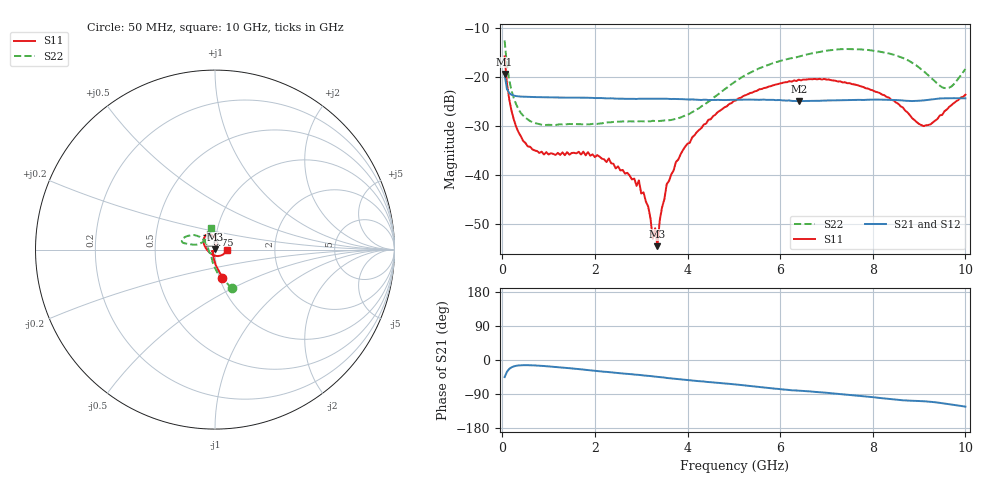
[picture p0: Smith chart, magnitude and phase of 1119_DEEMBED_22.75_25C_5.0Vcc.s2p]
!Hittite Microwave Corp.
!Digital Attenuator/PhaseShifter Rev 1.4.0
!Filename: C:\DATA\DATA\1119_DEEMBED_22.75_25C_5.0Vcc.s2p
!VNA ID: Agilent Technologies,N5224A,MY51441122,A.10.45.03
!Device type:
!2 Port Calibration.
!Temp(C): 25
!Lot Number:
!Serial Number:
!Operator:
!Misc:
!Attenuator:  22.750
# GHZ S DB R 50.0
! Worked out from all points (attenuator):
!   200 points, 50 MHz to 10 GHz, reference 50 ohm
!   highest |S21| = -19.44 dB at 50 MHz (marker M1); lowest = -25.0 dB at 6.4 GHz (marker M2)
!   lowest |S11| = -54.5 dB at 3.35 GHz (marker M3), VSWR 1.00, Z = 49.9 + j0.176 ohm
!   |S11| at or under -10 dB: start of sweep to end of sweep
!   |S22| runs from -29.8 to -12.6 dB; largest |S21 - S12| = 0.00016
!   S11 on the Smith chart (normalised r, x): 50 MHz: 1.03, -0.33; 6.75 GHz: 0.90, +0.15; 10 GHz: 1.14, -0.01
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0.05  -15.83 -75.3  -19.44 -45.1  -19.45 -45.1  -12.60 -66.6
0.1  -21.34 -87.5  -22.49 -31.2  -22.48 -31.2  -17.56 -83.5
0.2  -26.97 -99.7  -23.67 -19.3  -23.68 -19.2  -22.84 -100.2
0.45  -33.09 -117.7  -24.06 -13.7  -24.06 -13.7  -27.92 -120.8
0.9  -35.84 -137.5  -24.17 -15.9  -24.17 -15.9  -29.82 -135.1
1.75  -35.25 -145.1  -24.27 -25.3  -24.27 -25.3  -29.67 -139.8
2.95  -41.13 -130.7  -24.48 -39.3  -24.49 -39.4  -29.08 -158.8
3.15  -46.46 -133.5  -24.49 -41.7  -24.49 -41.8  -29.08 -164.8
3.25  -53.04 -163.3  -24.46 -43.2  -24.47 -43.2  -28.97 -167.5
3.3  -50.88 163.5  -24.48 -43.9  -24.49 -43.9  -29.03 -169.2
3.35  -54.53 109.9  -24.49 -44.5  -24.50 -44.5  -29.07 -170.8
3.4  -49.27 126.3  -24.48 -45.0  -24.49 -45.1  -29.01 -172.2
3.55  -41.89 90.1  -24.48 -47.4  -24.48 -47.4  -28.91 -177.6
3.9  -34.94 77.1  -24.57 -51.8  -24.58 -51.8  -28.11 168.1
5.05  -24.82 87.1  -24.70 -64.6  -24.71 -64.7  -20.85 139.4
6.4  -20.59 111.5  -24.96 -80.8  -24.97 -80.9  -15.90 150.6
6.7  -20.50 117.8  -24.88 -83.6  -24.90 -83.5  -15.20 154.5
6.75  -20.44 118.2  -24.89 -84.1  -24.90 -84.1  -15.12 155.1
8.35  -24.26 160.3  -24.71 -102.7  -24.71 -102.7  -15.25 168.2
9.1  -30.06 -125.9  -24.82 -108.9  -24.83 -108.9  -18.88 166.2
9.6  -26.67 -44.9  -24.38 -115.9  -24.39 -115.8  -22.32 133.3
10  -23.66 -2.1  -24.40 -123.1  -24.41 -123.1  -18.41 99.6
